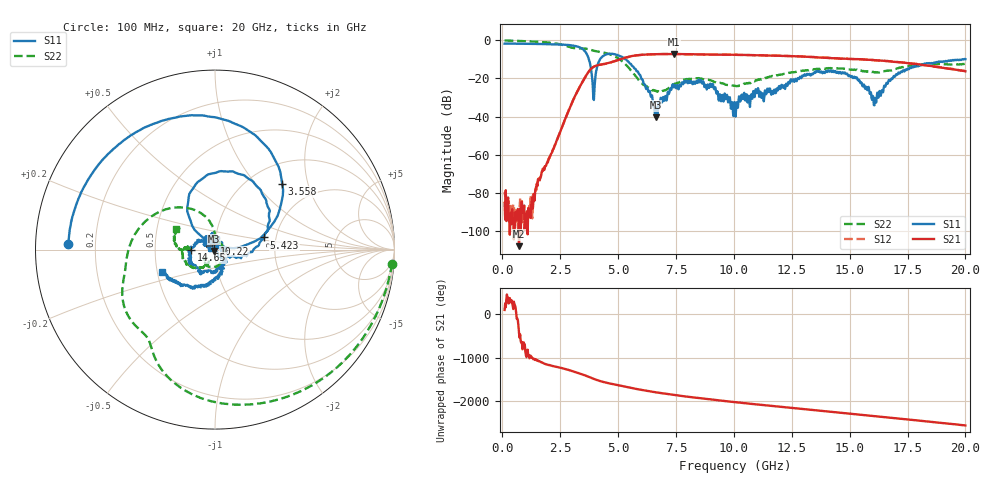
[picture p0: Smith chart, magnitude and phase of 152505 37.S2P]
!  2-Port S-parameters saved by WinCal
! VAR MeasName=S-Parameters (CALIBRATED_DATA) read from VNA (N5230C)
! VAR MeasDate=4/10/2015 9:32:10 AM
! VAR NAME=152505 37
! VAR FILENAME=152505 37.S2P
! VAR DATE=4/10/2015 9:32:10 AM
! VAR PHYS_PORTS=1,2
# Hz S DB R 50
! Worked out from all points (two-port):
!   801 points, 100 MHz to 20 GHz, reference 50 ohm
!   highest |S21| = -7.19 dB at 7.413 GHz (marker M1); lowest = -107.9 dB at 721.9 MHz (marker M2)
!   |S21| within 3 dB of the highest: 5.023 GHz to 15.78 GHz (10.76 GHz wide, 103 % of centre); 15.81942 GHz to 15.8225 GHz (3.083 MHz wide, 0.0195 % of centre)
!   lowest |S11| = -40.3 dB at 6.617 GHz (marker M3), VSWR 1.02, Z = 49.4 - j0.737 ohm
!   |S11| at or under -10 dB: 3.739 GHz to 4.22 GHz (480.2 MHz wide, 12.1 % of centre); 5.325 GHz to 19.86 GHz (14.53 GHz wide, 115 % of centre); 19.89382 GHz to 19.93244 GHz (38.62 MHz wide, 0.194 % of centre)
!   |S22| runs from -27.0 to -0.1 dB; largest |S21 - S12| = 0.0062
!   S11 on the Smith chart (normalised r, x): 100 MHz: 0.10, +0.02; 3.558 GHz: 1.38, +1.39; 5.423 GHz: 1.73, +0.25; 10.22 GHz: 0.99, +0.07; 14.65 GHz: 0.76, -0.00; 20 GHz: 0.53, -0.15
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1e8  -1.75 177.6  -85.23 89.5  -79.51 -66.0  -0.08 -4.6
7.21875e8  -1.80 162.7  -107.88 -74.0  -93.73 95.7  -0.34 -29.3
1.418375e9  -1.90 145.3  -79.35 23.9  -80.10 46.0  -0.68 -57.5
2.7865e9  -2.38 100.1  -39.12 168.0  -39.09 168.3  -3.08 -117.7
3.43325e9  -4.27 58.0  -22.43 57.8  -22.43 58.1  -4.25 -137.3
3.557625e9  -5.61 44.3  -19.75 34.7  -19.75 34.9  -4.33 -143.2
3.955625e9  -31.28 109.4  -13.81 -49.4  -13.81 -49.2  -5.47 -162.5
4.3785e9  -8.06 101.9  -12.45 -120.7  -12.48 -120.9  -6.44 177.9
5.42325e9  -11.03 14.0  -8.76 120.0  -8.75 120.0  -13.88 108.4
6.61725e9  -40.32 -129.3  -7.28 4.9  -7.26 4.8  -26.31 60.2
6.741625e9  -32.51 -166.1  -7.24 -5.4  -7.24 -5.6  -26.78 42.5
7.41325e9  -24.68 151.5  -7.19 -56.6  -7.19 -56.7  -22.95 -47.4
8.582375e9  -20.82 100.8  -7.40 -134.5  -7.36 -134.7  -20.08 -121.0
1.005e10  -34.42 129.1  -7.57 139.0  -7.60 138.9  -23.82 -127.3
1.022412e10  -29.36 98.5  -7.64 129.1  -7.64 129.5  -23.80 -124.0
1.201512e10  -25.51 -11.3  -8.15 32.2  -8.13 32.3  -18.03 -127.5
1.338325e10  -17.56 -108.6  -8.80 -39.8  -8.74 -39.5  -15.28 -148.4
1.465188e10  -17.47 -179.5  -9.62 -104.3  -9.57 -104.2  -14.76 -175.5
1.604488e10  -33.87 78.2  -10.38 -177.7  -10.39 -177.9  -16.75 177.9
1.669162e10  -20.79 -54.2  -10.96 147.6  -10.93 147.4  -15.91 -177.6
1.77115e10  -13.81 -101.6  -12.25 92.4  -12.18 92.0  -13.18 171.8
2e10  -9.88 -156.8  -16.22 -34.1  -16.19 -34.1  -12.27 151.8
